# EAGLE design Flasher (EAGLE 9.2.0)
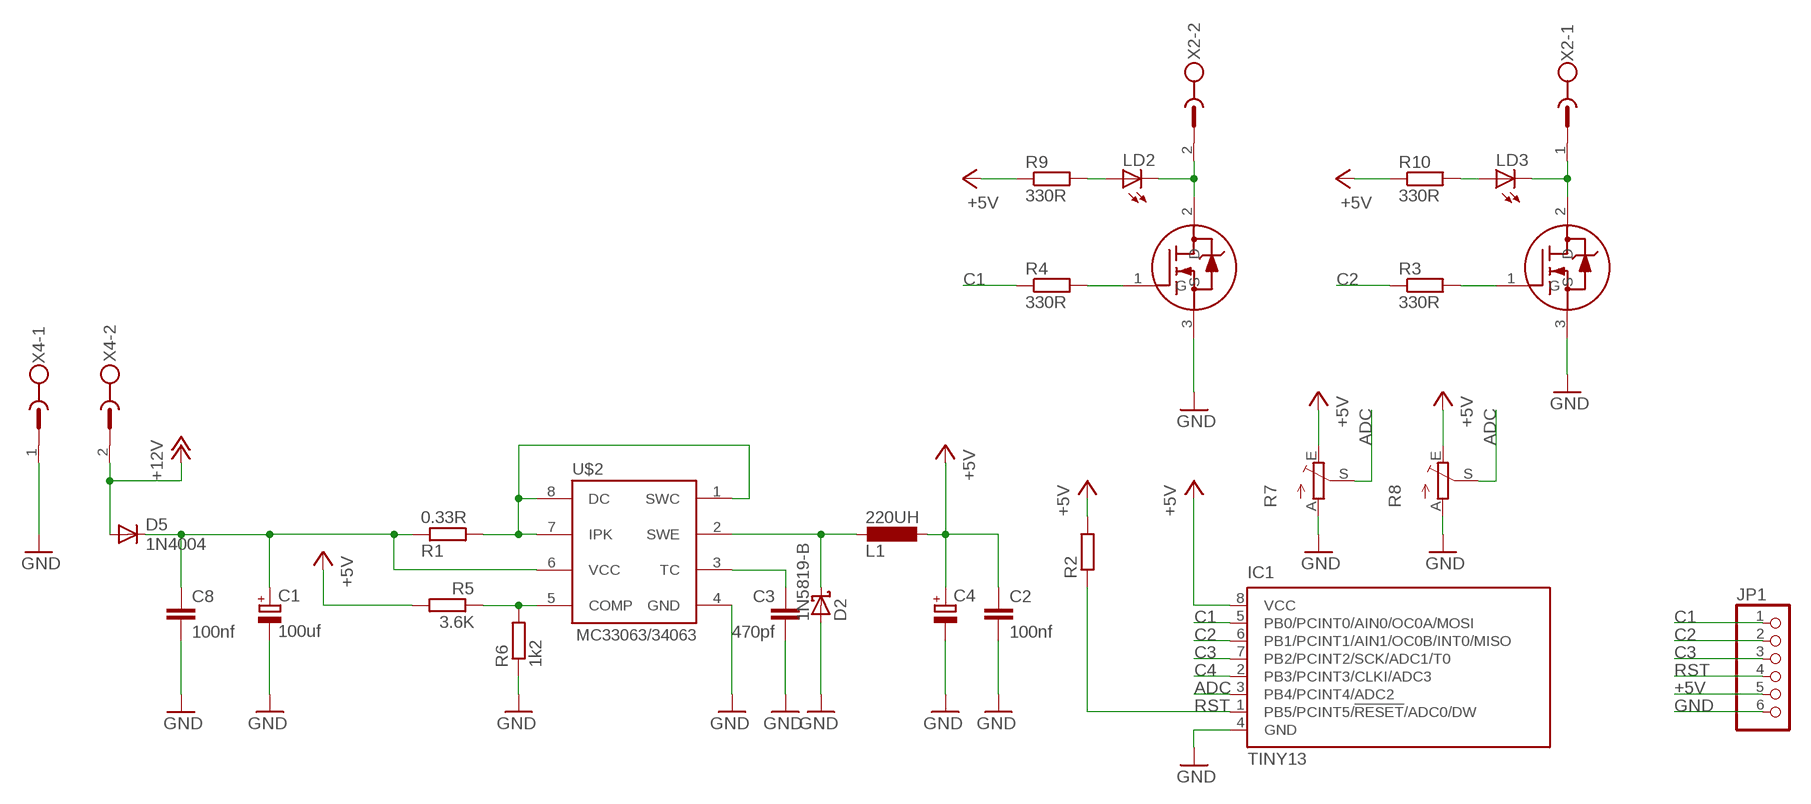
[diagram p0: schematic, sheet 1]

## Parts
C1  100uf  CPOL-EUE2-5  [E2-5]
C2  100nf  C-EUC0805K  [C0805K]
C3  470pf  C-EUC0805K  [C0805K]
C4  CPOL-EUE2.5-5  [E2,5-5]
C8  100nf  C-EUC0805K  [C0805K]
D2  1N5819-B  [DO41-7.6]
D5  1N4004  [DO41-10]
IC1  TINY13  TINY13-20SSU  [8S1]
JP1  PINHD-1X6  [1X06]
L1  220UH  L-EUL5650M  [L5650M]
LD2  LED3MM  [LED3MM]
LD3  LED3MM  [LED3MM]
R1  0.33R  R-EU_M0805  [M0805]
R2  R-EU_M0805  [M0805]
R3  330R  R-EU_M0805  [M0805]
R4  330R  R-EU_M0805  [M0805]
R5  3.6K  R-EU_M0805  [M0805]
R6  1k2  R-EU_M0805  [M0805]
R7  TRIM_EU-B25U  [B25U]
R8  TRIM_EU-B25P  [B25P]
R9  330R  R-EU_M0805  [M0805]
R10  330R  R-EU_M0805  [M0805]
U$1  20N03  [DPAK]
U$2  MC33063  MC33063/MC34063D  [SO08]
U$3  20N03  [DPAK]
X2  MSTBV2  [MSTBV2]
X4  MSTBV2  [MSTBV2]

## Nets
+5V: C2.1 C4.+ IC1.8(VCC) JP1.5 L1.1 R2.2 R5.2 R7.E R8.E R9.1 R10.1
+12V: D5.A X4.2
ADC: IC1.3(PB4/PCINT4/ADC2) R7.S R8.S
C1: IC1.5(PB0/PCINT0/AIN0/OC0A/MOSI) JP1.1 R4.1
C2: IC1.6(PB1/PCINT1/AIN1/OC0B/INT0/MISO) JP1.2 R3.1
C3: IC1.7(PB2/PCINT2/SCK/ADC1/T0) JP1.3
C4: IC1.2(PB3/PCINT3/CLKI/ADC3)
GND: C1.- C2.2 C3.2 C4.- C8.2 D2.A IC1.4(GND) JP1.6 R6.1 R7.A R8.A U$1.3(S) U$2.4(GND) U$3.3(S) X4.1
N$1: LD2.K(C) U$1.2(D) X2.2
N$2: R1.2 U$2.1(SWC) U$2.7(IPK) U$2.8(DC)
N$3: C3.1 U$2.3(TC)
N$4: R4.2 U$1.1(G)
N$6: LD3.K(C) U$3.2(D) X2.1
N$7: R3.2 U$3.1(G)
N$8: R5.1 R6.2 U$2.5(COMP)
N$9: D2.C L1.2 U$2.2(SWE)
N$10: C1.+ C8.1 D5.C R1.1 U$2.6(VCC)
N$13: LD2.A R9.2
N$14: LD3.A R10.2
RST: IC1.1(PB5/PCINT5/!RESET!/ADC0/DW) JP1.4 R2.1

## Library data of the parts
C1 C4 = rcl:CPOL-EU: POLARIZED CAPACITOR, European symbol; SPICEPREFIX: C
C2 C3 C8 = rcl:C-EU: CAPACITOR, European symbol
D2 = diode:1N581*: 1.0A SCHOTTKY BARRIER RECTIFIER
D5 = diode:1N4004: DIODE
IC1 = atmel:TINY13: 8-bit AVR Microcontroller with 1K Bytes In-System Programmable Flash Source: http://www.atmel.com/dyn/resources/prod_documents/2535S.pdf; MPN: ATTINY13-20SSU; OC_FARNELL: 1455133; OC_NEWARK: 58M3771
JP1 = pinhead:PINHD-1X6: PIN HEADER
L1 = rcl:L-EU: INDUCTOR, European symbol
LD2 LD3 = led:LED: LED
R1-R5 R9 R10 = rcl:R-EU_: RESISTOR, European symbol
R6 = rcl:R-EU_: RESISTOR, European symbol; SPICEPREFIX: R
R7 R8 = pot:TRIM_EU-: POTENTIOMETER
U$1 U$3 = 20n03:20N03
U$2 = adafruit:MC33063/MC34063: MC33063 and MC34063 Basic DC/DC converter with internal power-NPN transistor, 100KHz, 1.5A peak switch current. 3-40 input/output.
X2 X4 = con-phoenix-500:MSTBV2: PHOENIX; OC_FARNELL: unknown; OC_NEWARK: unknown

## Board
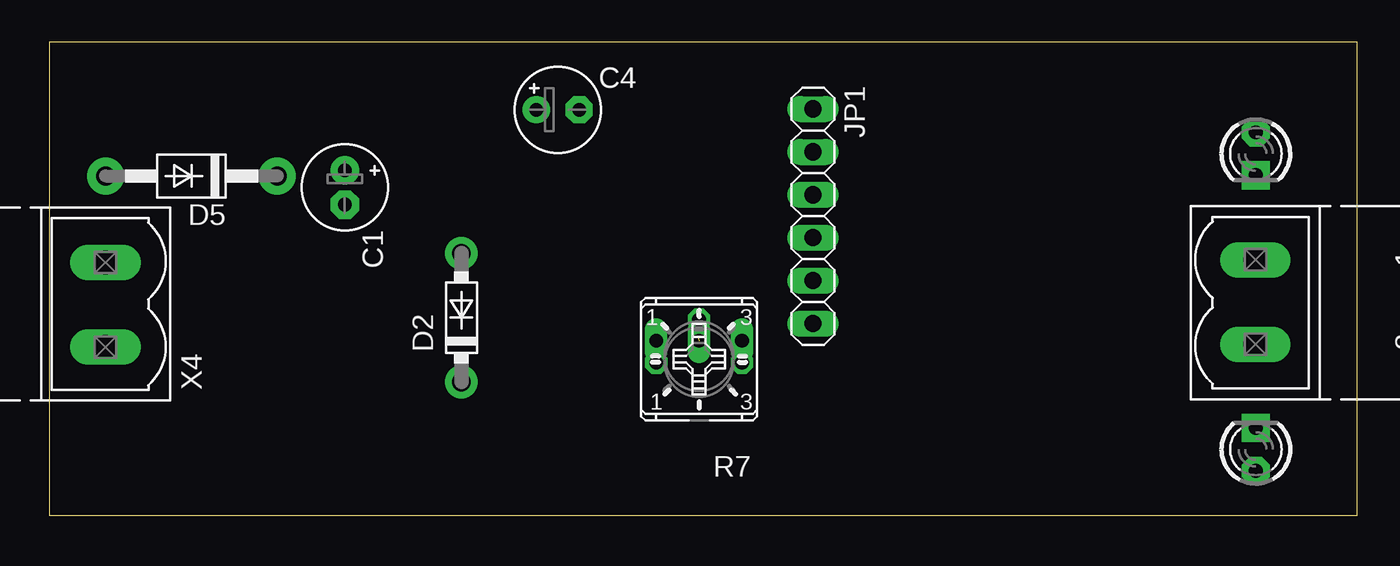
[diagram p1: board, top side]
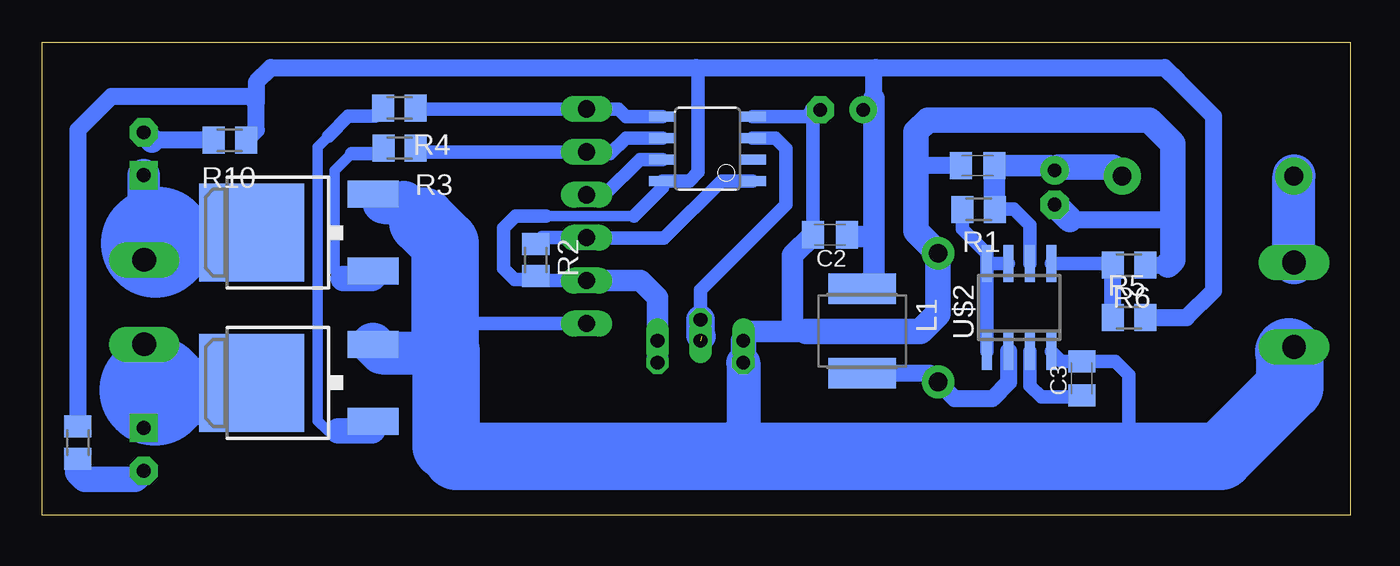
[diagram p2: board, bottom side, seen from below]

Size 77.4 x 28 mm. Coordinates in mm from the lower left corner, seen from the top.
Outline: 0,0 77.4,0 77.4,28 0,28 0,0
Copper layers (1*16): Top 0.035mm / dielectric 1.5mm / Bottom 0.035mm
Design rules "default": minimum track width 10mil, minimum drill 24mil, track to track 8mil, track to pad 8mil, pad to pad 8mil, via to via 8mil, smd to smd 8mil, copper to edge 40mil, drill to drill 8mil, minimum pad ring 10mil, minimum via ring 8mil, stop-mask expansion 4mil, vias tented up to drill 0mil, thermal gap 10mil

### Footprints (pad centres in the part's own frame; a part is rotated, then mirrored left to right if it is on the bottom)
E2-5 = drill 0.813 pad 1.676: + -1.016,0 | drill 0.813 pad 1.676 octagon: - 1.016,0
C0805K = smd 1.3 x 1.6: 1 -1,0; 2 1,0
E2,5-5 = drill 0.813 pad 1.6: + -1.27,0 | drill 0.813 pad 1.6 octagon: - 1.27,0
DO41-7.6 = drill 1.1 pad 1.93: A 3.81,0; C -3.81,0
DO41-10 = drill 1.118 pad 2.184: A 5.08,0; C -5.08,0
8S1 = smd 0.6 x 1.6: 1 -1.905,-2.654; 2 -0.645,-2.654; 3 0.625,-2.654; 4 1.895,-2.654; 5 1.905,2.654; 6 0.635,2.654; 7 -0.635,2.654; 8 -1.905,2.654
1X06 = drill 1.016 long: 1 -6.35,0; 2 -3.81,0; 3 -1.27,0; 4 1.27,0; 5 3.81,0; 6 6.35,0
L5650M = smd 1.8 x 4: 1 -2.5,0; 2 2.5,0
LED3MM = drill 0.813 pad 1.676 octagon: A -1.27,0 | drill 0.813 pad 1.676 square: K 1.27,0
M0805 = smd 1.3 x 1.6: 1 -0.95,0; 2 0.95,0
B25U = drill 0.813 long: A 2.54,-0.889; E -2.54,-0.889; S 0,-0.889
B25P = drill 0.813 octagon: A -2.54,0; E 2.54,0; S 0,2.54
DPAK = smd 1.6 x 3: 1 -2.28,-4.8; 3 2.28,-4.8 | smd 5.8 x 6.2: 2 0,2.38
SO08 = smd 0.6 x 2.2: 1 -1.905,-2.6; 2 -0.635,-2.6; 3 0.635,-2.6; 4 1.905,-2.6; 5 1.905,2.6; 6 0.635,2.6; 7 -0.635,2.6; 8 -1.905,2.6
MSTBV2 = drill 1.397 long: 1 -2.5,0; 2 2.5,0

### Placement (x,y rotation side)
C1  17.5,19.4 270 top
C2  30.8,16.6 180 bottom
C3  15.9,8.1 90 bottom
C4  30.1,24 0 top
C8  22.06,20.7 180 bottom
D2  24.4,11.7 90 top
D5  8.43,20.08 180 top
IC1  38.05,21.7 90 bottom
JP1  45.2,17.7 270 top
L1  28.9,10.9 270 bottom
LD2  71.4,3.9 90 top
LD3  71.4,21.4 270 top
R1  22,18.1 180 bottom
R2  48.2,15.1 270 bottom
R3  56.26,21.73 180 bottom
R4  56.27,24.11 180 bottom
R5  13.1,11.7 0 bottom
R6  13.1,14.8 180 bottom
R7  38.46,9.44 180 top
R8  38.46,9.04 0 top
R9  75.3,4.3 270 bottom
R10  66.3,22.2 180 bottom
U$1  62.63,7.84 90 bottom
U$2  19.6,12.3 0 bottom
U$3  62.63,16.73 90 bottom
X2  71.37,12.62 270 top
X4  3.35,12.46 90 top

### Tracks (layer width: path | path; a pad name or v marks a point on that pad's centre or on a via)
+5V
  Bottom 0.61: 42.4,17.7 47.6,17.7
  Bottom 0.813: 28.3,19.4 28.2,19.5 | 38.7,26.5 38.6,26.4 38.6,20.3 39.11,19.79 IC1.8 40.7,19.4 42.4,17.7 | JP1.5 47.94,13.89 R2.2 48.4,13.95 49.45,13.95 50.1,14.6 50.1,17 49.4,17.7 47.6,17.7
  Bottom 1: R5.2 9.7,11.7 8.1,13.3 8.1,23.6 10.2,25.7
  Bottom 1.016: 64.73,24.43 64.73,25.63 63.86,26.5 38.7,26.5 28.1,26.5 | 64.73,24.43 65.1,24.8 73.3,24.8 75.3,22.8 R9.1 | 10.2,25.7 11,26.5 28.1,26.5 | 28.2,24.7 28.2,26.4 28.1,26.5 | C4.+ 28.73,23.9 28.2,23.9 | R10.1 64.73,22.82 64.73,24.43
  Bottom 1.27: 28.2,16.5 28.2,19.5 28.2,23.9 28.2,24.7 | 28.2,16.5 28.2,14.1 L1.1 | C2.1 29.7,16.5 28.2,16.5 | R8.E R7.E 41,12.9 41.99,13.89 JP1.5
+12V
  Bottom 2.54: X4.2 D5.A
ADC  (1 unrouted)
  Bottom 0.813: IC1.3 34.02,22.32 33.4,21.7 33.4,18.4 38.46,13.34 R8.S
  Bottom 1.676: 38.4,10.59 38.46,10.65 R8.S
C1
  Bottom 0.813: IC1.5 42.85,23.6 43.3,24.05 JP1.1 55.26,24.05 R4.1
C2
  Bottom 0.813: IC1.6 42.87,22.33 43.8,21.4 45.09,21.4 JP1.2 55.09,21.51 R3.1
C3
  Bottom 0.813: IC1.7 42.04,21.06 44.13,18.97 JP1.3
GND
  Bottom 0.813: U$3.3 57.33,18.51 57.2,18.51 | U$2.4 17.09,9.1 C3.2 13.9,9.1 13.1,8.3 13.1,3.5 | C2.2 31.8,24 32.21,23.59 IC1.4 | JP1.6 53.13,11.35 53.58,11.8
  Bottom 1: R6.1 10.8,14.8 | 23.1,20.74 C8.2
  Bottom 1.016: X4.1 2.76,9.96 | C8.2 25.6,20.7 25.7,20.8 | 16.62,17.5 10.5,17.5 | C4.- 31.8,24
  Bottom 1.27: 35.92,5.32 34.1,3.5 | 53.41,9.7 53.5,9.7 | 53.38,12 53.58,11.8 | 32.22,10.87 33,10.87 | 33,10.87 35.38,10.87 R7.A | 33,10.87 33,15.4 C2.2
  Bottom 1.5: C1.- 16.62,17.5 | 10.8,14.8 10.5,15.1 10.5,17.5 10.5,22 11.9,23.4 25,23.4 25.7,22.7 25.7,20.8 25.7,16.81 D2.A 24.4,11.9 25.43,10.87 32.22,10.87 | R7.A R8.A
  Bottom 1.676: 42.46,3.96 42,3.5
  Bottom 2: R8.A 35.92,5.32
  Bottom 2.54: U$1.3 57.33,9.62 53.58,9.62 | 54.9,17.4 56.01,18.51 57.2,18.51
  Bottom 3: 3.65,9.66 X4.1
  Bottom 3.81: 53.58,9.62 53.5,9.7 | 53.5,4.1 52.9,3.5
  Bottom 4: 53.5,9.7 53.5,4.1 53,4.1 | 52.9,3.5 42,3.5 34.1,3.5 13.1,3.5 7.7,3.5 3.6,7.6 3.6,9.61 3.65,9.66 | 53.58,9.62 53.58,11.8 53.58,16.08 54.9,17.4
N$1
  Bottom 1.93: 70.8,7.4 70.8,9.05 71.37,9.62 X2.2 | LD2.K 71.4,6.68 70.74,7.34
  Bottom 4: 70.74,7.34 65.51,7.34 U$1.2
  Bottom 6.452: 70.8,7.4 70.74,7.34
N$2
  Bottom 0.813: U$2.7 U$2.8 | R1.2 22.95,16.95 21.5,15.51 U$2.8 | U$2.8 U$2.1
N$3
  Bottom 0.813: U$2.3 18.96,7.67 18.3,7 16,7 C3.1
N$4
  Bottom 0.61: 60.2,22.7 60.45,22.45 61.1,21.8 61.1,5.6 60.5,5 59.9,5
  Bottom 0.813: R4.2 57.72,23.61 59.29,23.61 60.45,22.45
  Bottom 1.5: 59.9,5 57.89,5 57.83,5.06 U$1.1
N$6
  Bottom 1.778: 70.7,16.1 70.7,15.8 70.7,15.29 70.87,15.12 X2.1
  Bottom 1.93: LD3.K 71.4,16.5 70.7,15.8
  Bottom 4: 70.57,16.23 65.51,16.23 U$3.2
  Bottom 6.452: 70.7,16.1 70.57,16.23
N$7
  Bottom 0.61: 59.1,21.4 60.1,20.4 60.1,14.5 59.6,14
  Bottom 0.813: 59.1,21.4 57.38,21.4 57.21,21.57 R3.2
  Bottom 1.5: 59.6,14 57.88,14 57.83,14.05 U$3.1
N$8
  Bottom 0.813: R6.2 14.15,14.9 U$2.5
  Bottom 1.016: R5.1 R6.2
N$9
  Bottom 1: U$2.2 20.23,7.87 21.2,6.9 23.41,6.9 D2.C 24.91,8.4 L1.2
N$10
  Bottom 0.813: U$2.6 18.96,17.16 19.91,18.11 R1.1
  Bottom 1.27: 14.05,20.62 D5.C | C1.+ 17.78,20.7 C8.1 R1.1
  Bottom 1.5: C1.+ 17.3,20.62 14.05,20.62
N$13
  Bottom 1.016: R9.2 75.3,2.53
  Bottom 1.5: 75.3,2.53 74.9,2.13 71.9,2.13 LD2.A
N$14
  Bottom 1.016: R10.2 70.93,22.2 LD3.A
  Bottom 1.422: LD3.A 70.9,22.17
RST
  Bottom 0.813: IC1.1 37.21,19.79 40.6,16.4 45.17,16.4 JP1.4 47.82,16.43 R2.1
